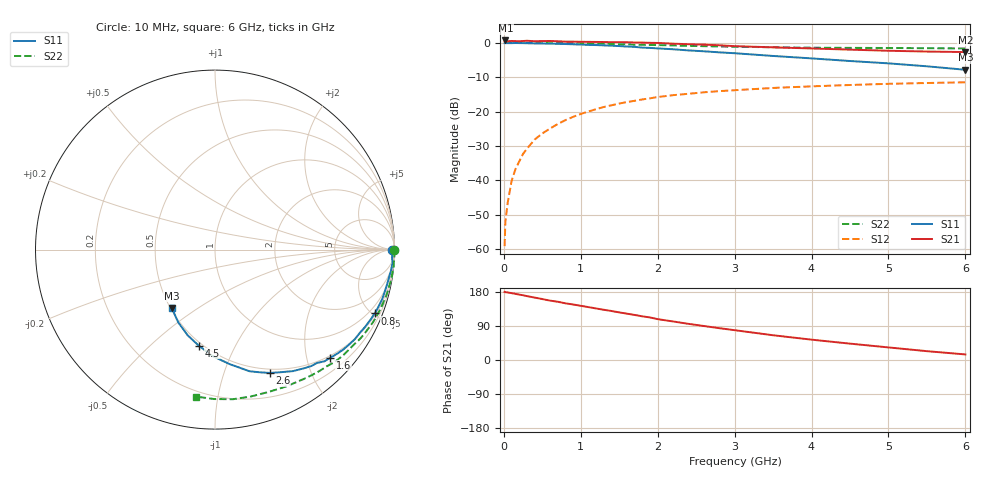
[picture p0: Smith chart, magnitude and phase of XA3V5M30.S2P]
! SIEMENS Discrete & RF Semiconductors
! BFY180
! Si NPN RF Bipolar Junction Transistor in MICRO-X
! VCE = 3.5 V  IC = 0.3 mA
! Common Emitter S-Parameters:  May  1997
# GHz  S  MA  R  50
!  f  S11  S21  S12  S22
! GHz  MAG  ANG  MAG  ANG  MAG  ANG  MAG  ANG
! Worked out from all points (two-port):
!   36 points, 10 MHz to 6 GHz, reference 50 ohm
!   highest |S21| = 0.67 dB at 20 MHz (marker M1); lowest = -2.7 dB at 6 GHz (marker M2)
!   |S21| within 3 dB of the highest: start of sweep to 5.01 GHz
!   lowest |S11| = -7.9 dB at 6 GHz (marker M3), VSWR 2.36, Z = 25.4 - j19.7 ohm
!   |S11| at or under -10 dB: nowhere
!   |S22| runs from -1.7 to 0.0 dB; largest |S21 - S12| = 1.1
!   S11 on the Smith chart (normalised r, x): 10 MHz: open; 800 MHz: 0.59, -5.13; 1.6 GHz: 0.46, -2.46; 2.6 GHz: 0.46, -1.44; 4.5 GHz: 0.48, -0.73; 6 GHz: 0.51, -0.39
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0.01  0.9871 -0.2  1.053 179.9  0.0011 89.6  0.9999 -0.2
0.02  0.9874 -0.5  1.08 179.0  0.0025 87.3  0.9999 -0.4
0.05  0.9879 -1.2  1.052 178.3  0.0047 90.9  0.9995 -1.0
0.1  0.9876 -2.7  1.062 176.4  0.0097 90.1  0.9999 -2.1
0.15  0.9914 -4.3  1.057 174.6  0.0144 87.4  0.9996 -3.1
0.25  0.9875 -7.1  1.06 170.9  0.0242 85.3  0.9997 -5.3
0.4  0.9787 -11.0  1.053 164.8  0.039 81.5  0.9968 -8.3
0.5  0.9745 -13.9  1.059 160.8  0.048 78.7  0.994 -10.4
0.6  0.9716 -16.4  1.061 156.7  0.0565 76.5  0.9906 -12.5
0.8  0.9583 -21.8  1.039 149.6  0.0749 71.7  0.9846 -16.6
1.1  0.9308 -29.8  1.03 139.5  0.1 65.2  0.9728 -22.6
1.6  0.881 -43.1  1.018 122.3  0.1372 54.4  0.946 -32.4
1.9  0.8416 -50.5  0.998 112.3  0.1556 48.5  0.9291 -37.8
2  0.8273 -53.0  0.994 107.8  0.1624 46.7  0.9254 -39.6
2.2  0.8045 -57.3  0.97 101.7  0.1728 43.0  0.9155 -43.0
2.6  0.7516 -66.1  0.94 89.7  0.1902 36.5  0.8923 -49.3
3  0.7042 -74.2  0.892 78.7  0.204 30.3  0.8743 -55.5
3.5  0.6427 -82.8  0.858 65.3  0.2201 24.0  0.8599 -62.3
4  0.5925 -91.5  0.826 53.7  0.2322 17.8  0.8477 -69.2
4.5  0.5426 -99.6  0.794 43.2  0.243 12.3  0.8424 -76.2
5.5  0.4544 -116.8  0.745 23.3  0.2597 1.6  0.8327 -90.3
6  0.4044 -126.6  0.732 14.7  0.266 -3.9  0.8257 -97.4
